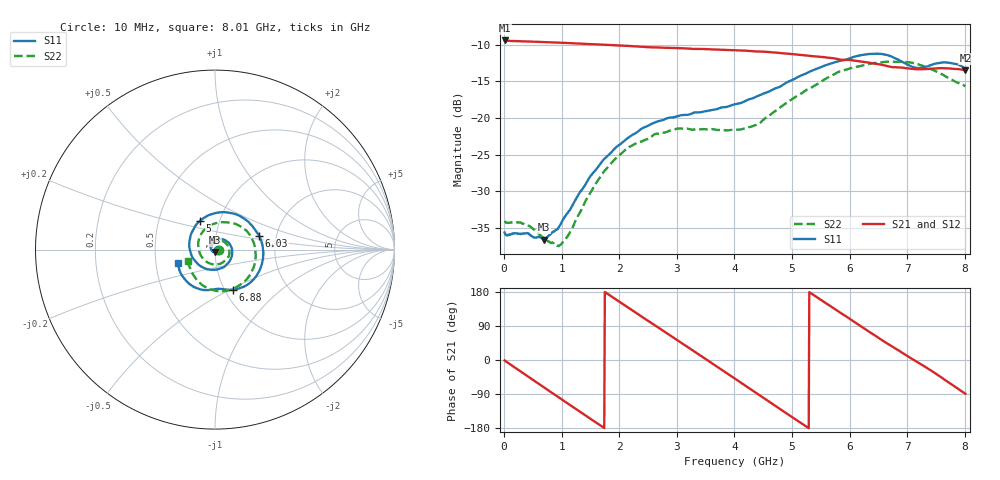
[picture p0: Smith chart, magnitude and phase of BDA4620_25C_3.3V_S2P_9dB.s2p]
!Agilent Technologies,E5071B,MY42404982,A.09.10
!Date: Wed May 06 08:50:18 2026
!Data & Calibration Information:
!Freq	S11:SOLT2(ON)	S21:SOLT2(ON)	S12:SOLT2(ON)	S22:SOLT2(ON)
# Hz S RI R 50
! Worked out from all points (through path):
!   801 points, 10 MHz to 8.01 GHz, reference 50 ohm
!   highest |S21| = -9.44 dB at 10 MHz (marker M1); lowest = -13.5 dB at 8.01 GHz (marker M2)
!   group delay of S21, straight-line fit = 280 ps
!   lowest |S11| = -36.6 dB at 700 MHz (marker M3), VSWR 1.03, Z = 49.8 - j1.45 ohm
!   |S11| at or under -10 dB: start of sweep to end of sweep
!   |S22| runs from -37.5 to -12.3 dB; largest |S21 - S12| = 0.0015
!   S11 on the Smith chart (normalised r, x): 10 MHz: 1.03, -0.00; 5 GHz: 0.81, +0.27; 6.03 GHz: 1.63, +0.26; 6.88 GHz: 1.10, -0.52; 8.01 GHz: 0.65, -0.10
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1e7  0.0165 -0.00117  0.3372 -0.00719  0.3374 -0.00735  0.0197 -0.00121
3.3e8  0.0127 -0.0102  0.2737 -0.1888  0.2741 -0.1895  0.0165 -0.00946
7e8  -0.00211 -0.0146  0.0967 -0.3143  0.0967 -0.3148  0.00296 -0.0148
9.8e8  -0.0175 -0.0066  -0.0664 -0.3188  -0.0663 -0.3192  -0.0107 -0.00843
1.35e9  -0.0249 0.0207  -0.2448 -0.2072  -0.245 -0.2075  -0.0188 0.0149
1.65e9  -0.0103 0.0461  -0.3117 -0.0531  -0.3123 -0.0532  -0.00914 0.0373
1.94e9  0.0193 0.0597  -0.2939 0.1061  -0.2942 0.1065  0.0148 0.0509
2.32e9  0.0659 0.0461  -0.1602 0.2618  -0.1604 0.2621  0.0531 0.0423
2.68e9  0.095 0.000886  0.0244 0.301  0.0246 0.3015  0.0773 0.011
3e9  0.0873 -0.0532  0.1797 0.2396  0.1802 0.2396  0.0791 -0.0293
3.39e9  0.0366 -0.1028  0.2866 0.0703  0.2871 0.07  0.0437 -0.0711
4.01e9  -0.0896 -0.0854  0.1885 -0.2195  0.1886 -0.2201  -0.0546 -0.0626
4.49e9  -0.1437 0.0241  -0.0413 -0.28  -0.0415 -0.2805  -0.0936 0.0218
5e9  -0.0824 0.1611  -0.2371 -0.134  -0.2376 -0.134  -0.0357 0.1293
5.35e9  0.0306 0.2082  -0.2624 0.0274  -0.2625 0.0276  0.0554 0.1523
6.03e9  0.2461 0.0759  -0.067 0.2382  -0.0669 0.2388  0.2157 0.0374
6.35e9  0.2645 -0.0668  0.0678 0.2274  0.0679 0.2277  0.2242 -0.065
6.68e9  0.18 -0.1962  0.1694 0.1469  0.17 0.1471  0.1758 -0.1663
6.88e9  0.1014 -0.2236  0.2042 0.0841  0.2045 0.0841  0.1228 -0.2078
7.18e9  0.019 -0.2181  0.2134 -0.0218  0.2137 -0.0218  0.019 -0.2319
7.55e9  -0.0909 -0.2186  0.1636 -0.1449  0.1635 -0.145  -0.0887 -0.1822
8.01e9  -0.2044 -0.0724  0.00369 -0.2114  0.00375 -0.212  -0.1507 -0.0654
